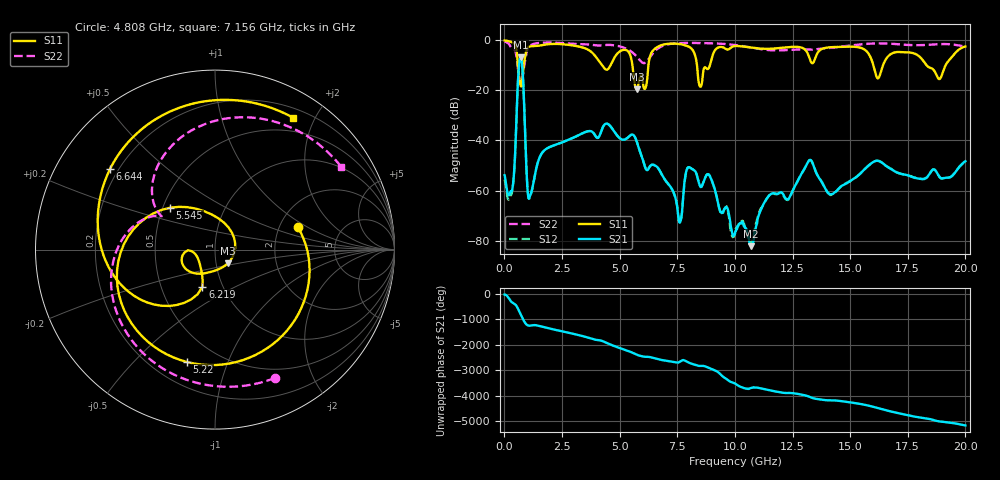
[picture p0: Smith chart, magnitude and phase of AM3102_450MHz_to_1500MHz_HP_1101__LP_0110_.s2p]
!Agilent Technologies,E8364B,MY43040894,A.07.50.67
!Agilent E8364B: A.07.50.67
!Date: Thursday, January 11, 2018 06:38:49
!Correction: S11(Full 2 Port(1,2))
!S21(Full 2 Port(1,2))
!S12(Full 2 Port(1,2))
!S22(Full 2 Port(1,2))
!S2P File: Measurements: S11, S21, S12, S22:
# Hz S  dB  R 50
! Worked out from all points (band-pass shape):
!   1601 points, 10 MHz to 20 GHz, reference 50 ohm
!   highest |S21| = -6.86 dB at 709.6 MHz (marker M1); lowest = -82.2 dB at 10.7 GHz (marker M2)
!   |S21| within 3 dB of the highest: 637.7 MHz to 772.2 MHz (134.5 MHz wide, 19.1 % of centre)
!   lowest |S11| = -19.6 dB at 5.745 GHz (marker M3), VSWR 1.23, Z = 56.8 - j8.9 ohm
!   |S11| at or under -10 dB: 5.556 GHz to 6.247 GHz (691.6 MHz wide, 11.7 % of centre); 8.357 GHz to 8.916 GHz (558.9 MHz wide, 6.47 % of centre); 18.32 GHz to 19.14 GHz (818.5 MHz wide, 4.37 % of centre)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
!   |S22| runs from -17.1 to -0.4 dB; largest |S21 - S12| = 0.001
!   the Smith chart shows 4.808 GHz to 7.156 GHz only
!   S11 on the Smith chart (normalised r, x): 4.808 GHz: 2.54, +0.81; 5.22 GHz: 0.34, -0.72; 5.545 GHz: 0.55, +0.29; 6.219 GHz: 0.80, -0.35; 6.644 GHz: 0.17, +0.33; 7.156 GHz: 0.32, +1.71
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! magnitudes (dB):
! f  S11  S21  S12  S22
! 10 MHz  -0.1  -53.9  -55.6  -0.4
! 347.3 MHz  -0.9  -59.3  -59.6  -3.4
! 709.6 MHz  -18.3  -6.9  -6.9  -16.9
! 1.097 GHz  -2.5  -62.6  -62.9  -2.2
! 3.346 GHz  -2.8  -37.3  -37.3  -1.5
! 4.808 GHz  -6.4  -37.0  -36.9  -2.1
! 5.22 GHz  -3.8  -39.6  -39.6  -3.1
! 5.545 GHz  -9.3  -37.6  -37.7  -4.8
! 5.745 GHz  -19.6  -40.5  -40.4  -6.5
! 6.219 GHz  -13.2  -51.7  -51.6  -8.0
! 6.644 GHz  -2.6  -50.7  -50.7  -3.4
! 6.682 GHz  -2.5  -51.2  -51.2  -3.2
! 7.156 GHz  -1.4  -57.9  -57.9  -1.5
! 7.619 GHz  -1.5  -72.7  -72.4  -1.1
! 7.956 GHz  -2.4  -50.8  -50.9  -1.0
! 8.493 GHz  -18.5  -58.3  -58.2  -1.1
! 10.01 GHz  -2.3  -77.2  -76.1  -1.9
! 10.7 GHz  -2.9  -82.2  -80.8  -2.9
! 13.34 GHz  -9.1  -48.4  -48.4  -3.7
! 14.18 GHz  -2.8  -61.5  -61.7  -3.0
! 16.68 GHz  -6.1  -50.9  -50.8  -1.3
! 20 GHz  -2.5  -48.3  -48.4  -2.4
